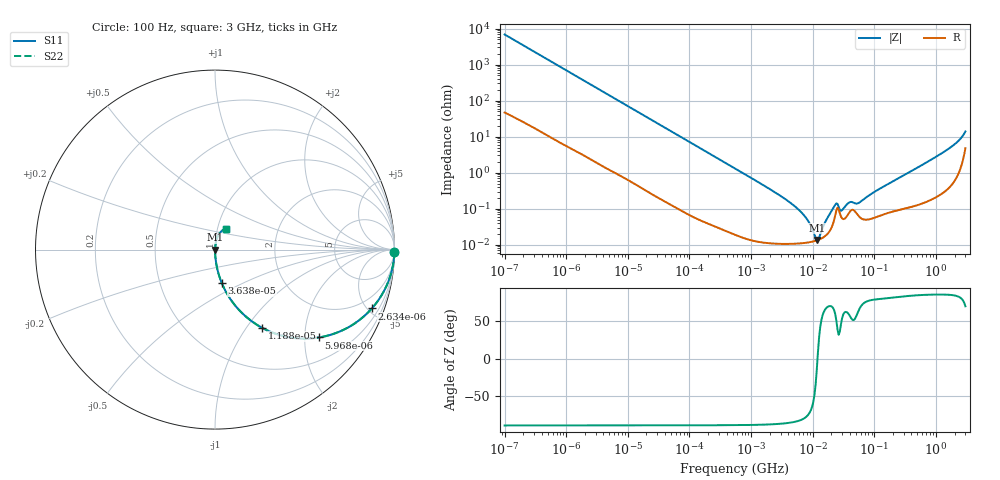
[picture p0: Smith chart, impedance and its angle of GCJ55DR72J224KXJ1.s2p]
!Murata Part Number: GCJ55DR72J224KXJ1
!These Parameters are Measured in Series Mode Connection
!Data Generated on Mar 13, 2026
!  o--ll--o
!Port1  Port2
!  o------o
!Operation Temp=25[degC], DC Bias Voltage=0[V]
!Freq. Start=100[Hz] Stop=3[GHz] 401[Steps]
# Hz S RI R 50
!Freq.(Hz) S11(Real) S11(Imag) S21(Real) S21(Imag) S12(Real) S12(Imag) S22(Real) S22(Imag)
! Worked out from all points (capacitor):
!   401 points, 100 Hz to 3 GHz, reference 50 ohm
!   read as one part in series: C = 231 nF near 109 Hz
!   lowest |Z| = 13.6 mohm at 11.63 MHz (marker M1)
!   series resonance near 11.96 MHz, so ESL is about 770 pH
!   S11 on the Smith chart (normalised r, x): 100 Hz: open; 2.634 kHz: 1.04, -5.31; 5.968 kHz: 1.02, -2.35; 11.88 kHz: 1.01, -1.19; 36.38 kHz: 1.00, -0.39; 3 GHz: 1.10, +0.26
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100  0.9997 -0.0145  0.00031 0.0145  0.00031 0.0145  0.9997 -0.0145
536  0.9935 -0.0767  0.00651 0.0767  0.00651 0.0767  0.9935 -0.0767
1788  0.9366 -0.2395  0.0634 0.2395  0.0634 0.2395  0.9366 -0.2395
2634  0.8737 -0.328  0.1263 0.328  0.1263 0.328  0.8737 -0.328
5968  0.58 -0.4893  0.42 0.4893  0.42 0.4893  0.58 -0.4893
11882  0.2623 -0.4355  0.7377 0.4355  0.7377 0.4355  0.2623 -0.4355
31977  0.0485 -0.2106  0.9515 0.2106  0.9515 0.2106  0.0485 -0.2106
36384  0.0382 -0.1872  0.9618 0.1872  0.9618 0.1872  0.0382 -0.1872
547723  0.00036 -0.0131  0.9996 0.0131  0.9996 0.0131  0.00036 -0.0131
4711951  0.000108 -0.0013  0.9999 0.0013  0.9999 0.0013  0.000108 -0.0013
7246509  0.000112 -0.000641  0.9999 0.000641  0.9999 0.000641  0.000112 -0.000641
9794414  0.000121 -0.00025  0.9999 0.00025  0.9999 0.00025  0.000121 -0.00025
1.163455e7  0.000132 -3.46e-05  0.9999 3.46e-05  0.9999 3.46e-05  0.000132 -3.46e-05
1.268047e7  0.000139 7.5e-05  0.9999 -7.5e-05  0.9999 -7.5e-05  0.000139 7.5e-05
1.641694e7  0.000182 0.000434  0.9998 -0.000434  0.9998 -0.000434  0.000182 0.000434
2.316512e7  0.00065 0.00111  0.9993 -0.00111  0.9993 -0.00111  0.00065 0.00111
2.999103e7  0.000534 0.00074  0.9995 -0.00074  0.9995 -0.00074  0.000534 0.00074
4.0536e7  0.000851 0.00127  0.9991 -0.00127  0.9991 -0.00127  0.000851 0.00127
5.478864e7  0.000643 0.00127  0.9994 -0.00127  0.9994 -0.00127  0.000643 0.00127
1.751444e8  0.000806 0.00499  0.9992 -0.00499  0.9992 -0.00499  0.000806 0.00499
1.443257e9  0.00479 0.0405  0.9952 -0.0405  0.9952 -0.0405  0.00479 0.0405
3e9  0.0602 0.1174  0.9398 -0.1174  0.9398 -0.1174  0.0602 0.1174
